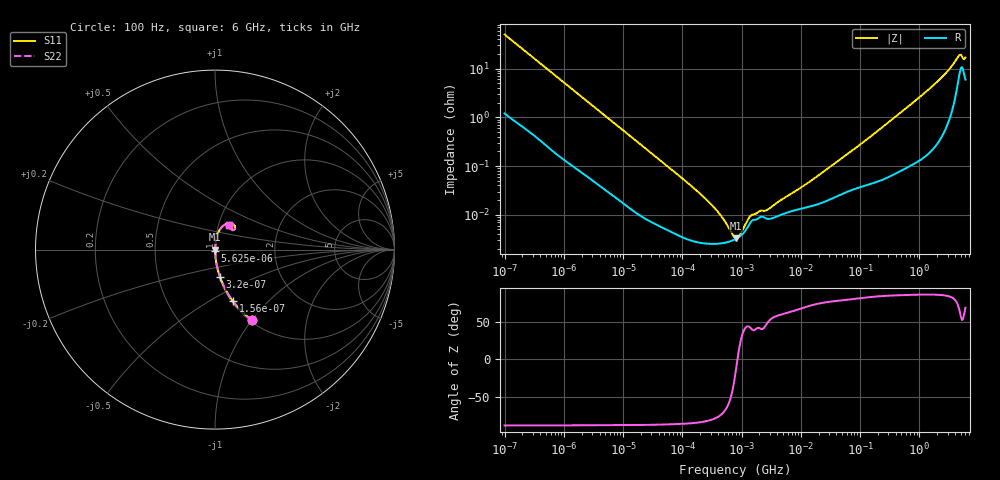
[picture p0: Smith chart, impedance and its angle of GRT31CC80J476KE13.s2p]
!Murata Part Number: GRT31CC80J476KE13
!These Parameters are Measured in Series Mode Connection
!Data Generated on Jun 19, 2026
!  o--ll--o
!Port1  Port2
!  o------o
!Operation Temp=25[degC], DC Bias Voltage=0[V]
!Freq. Start=100[Hz] Stop=6[GHz] 401[Steps]
# Hz S RI R 50
!Freq.(Hz) S11(Real) S11(Imag) S21(Real) S21(Imag) S12(Real) S12(Imag) S22(Real) S22(Imag)
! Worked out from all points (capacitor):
!   401 points, 100 Hz to 6 GHz, reference 50 ohm
!   read as one part in series: C = 31.6 uF near 109 Hz
!   lowest |Z| = 3.29 mohm at 810.1 kHz (marker M1)
!   series resonance near 851 kHz, so ESL is about 1.1 nH
!   S11 on the Smith chart (normalised r, x): 100 Hz: 1.02, -1.00; 156 Hz: 1.02, -0.64; 320 Hz: 1.01, -0.32; 5.625 kHz: 1.00, -0.02; 6 GHz: 1.12, +0.32
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100  0.2062 -0.3928  0.7938 0.3928  0.7938 0.3928  0.2062 -0.3928
156  0.0997 -0.2876  0.9003 0.2876  0.9003 0.2876  0.0997 -0.2876
320  0.0286 -0.154  0.9714 0.154  0.9714 0.154  0.0286 -0.154
717  0.00697 -0.0714  0.993 0.0714  0.993 0.0714  0.00697 -0.0714
2008  0.00141 -0.0261  0.9986 0.0261  0.9986 0.0261  0.00141 -0.0261
5625  0.000382 -0.00951  0.9996 0.00951  0.9996 0.00951  0.000382 -0.00951
40335  6.09e-05 -0.00137  0.9999 0.00137  0.9999 0.00137  6.09e-05 -0.00137
184852  2.72e-05 -0.000293  1 0.000293  1 0.000293  2.72e-05 -0.000293
432798  2.58e-05 -9.81e-05  1 9.81e-05  1 9.81e-05  2.58e-05 -9.81e-05
473344  2.62e-05 -8.37e-05  1 8.37e-05  1 8.37e-05  2.62e-05 -8.37e-05
774597  3.13e-05 -1.29e-05  1 1.29e-05  1 1.29e-05  3.13e-05 -1.29e-05
810067  3.22e-05 -6.8e-06  1 6.8e-06  1 6.8e-06  3.22e-05 -6.8e-06
1516199  7.69e-05 6.45e-05  0.9999 -6.45e-05  0.9999 -6.45e-05  7.69e-05 6.45e-05
2713602  8.29e-05 9.53e-05  0.9999 -9.53e-05  0.9999 -9.53e-05  8.29e-05 9.53e-05
1.555665e7  0.000152 0.000497  0.9998 -0.000497  0.9998 -0.000497  0.000152 0.000497
9.326766e7  0.000365 0.00255  0.9996 -0.00255  0.9996 -0.00255  0.000365 0.00255
3.124326e8  0.000671 0.00813  0.9993 -0.00813  0.9993 -0.00813  0.000671 0.00813
1.873145e9  0.00498 0.0493  0.995 -0.0493  0.995 -0.0493  0.00498 0.0493
3.505958e9  0.024 0.1063  0.976 -0.1063  0.976 -0.1063  0.024 0.1063
4.586474e9  0.0794 0.1471  0.9206 -0.1471  0.9206 -0.1471  0.0794 0.1471
5.245841e9  0.112 0.1147  0.888 -0.1147  0.888 -0.1147  0.112 0.1147
6e9  0.0767 0.1382  0.9233 -0.1382  0.9233 -0.1382  0.0767 0.1382
